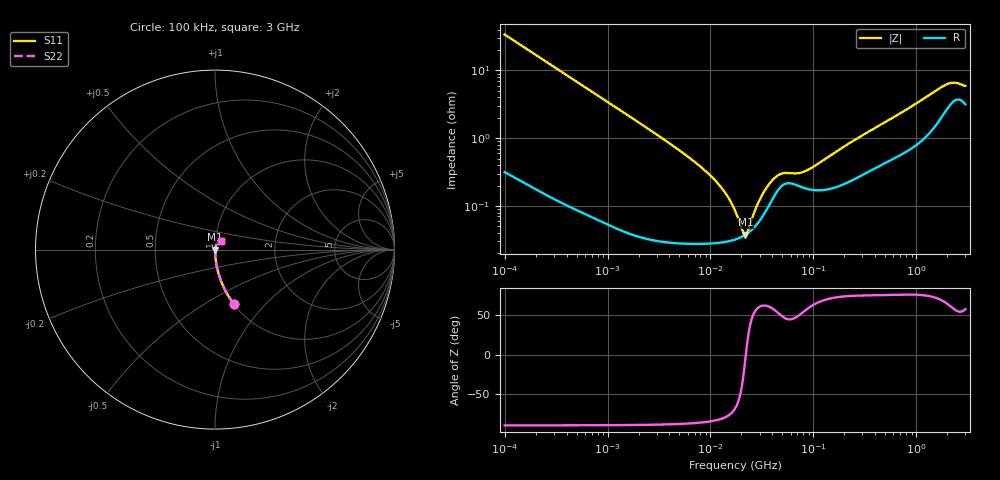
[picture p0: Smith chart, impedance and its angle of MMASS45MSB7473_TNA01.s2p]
! MMASS45MSB7473_TNA01  S-PARAMETER MODEL  ( Standard Model )
! Model Generated by TAIYO YUDEN Corporation (http://www.ty-top.com)
! Version 1.0
! TAIYO YUDEN Control No. 220601
! Copyright(c) 2013 TAIYO YUDEN CO.,LTD. All Rights Reserved.
! Product Description (link to TY-COMPAS)
! https://ds.yuden.co.jp/TYCOMPAS/or/detail?pn=MMASS45MSB7473KTNA01&u=M
! Products Name : Multilayer Ceramic Capacitors
! Characteristics :
!  Capacitance : 0.047 [uF] , Rated Voltage : 630 [V] , TCC : X7R
!  Case Size : 4.5 x 3.2 / 0.177 x 0.126 [mm/inch] , Thickness : 2.5 / 0.098 [mm/inch]
!  (Conditions: Temperature = 25 [degC] , DC Bias Voltage = 0 [V])
! External Node Assignments :
!  1  o---| |---o  2
! GND o---------o GND
! Frequency Range : 100kHz  -  3GHz  [ 401 STEP ]
# MHZ S RI R 50
! Freq[MHz].  S11 Real  S11 Imag  S21 Real  S21 Imag  S12 Real  S12 Imag  S22 Real  S22 Imag
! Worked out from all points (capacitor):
!   401 points, 100 kHz to 3 GHz, reference 50 ohm
!   read as one part in series: C = 46.7 nF near 105.3 kHz
!   lowest |Z| = 37.7 mohm at 21.84 MHz (marker M1)
!   series resonance near 22.07 MHz, so ESL is about 1.1 nH
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0.1  0.1059 -0.3031  0.8941 0.3031  0.8941 0.3031  0.1059 -0.3031
0.228123  0.0234 -0.1461  0.9766 0.1461  0.9766 0.1461  0.0234 -0.1461
0.562235  0.00451 -0.0608  0.9955 0.0608  0.9955 0.0608  0.00451 -0.0608
3.161081  0.000416 -0.0107  0.9996 0.0107  0.9996 0.0107  0.000416 -0.0107
6.504802  0.0003 -0.00489  0.9997 0.00489  0.9997 0.00489  0.0003 -0.00489
10.34438  0.000287 -0.00265  0.9997 0.00265  0.9997 0.00265  0.000287 -0.00265
14.09348  0.000298 -0.00149  0.9997 0.00149  0.9997 0.00149  0.000298 -0.00149
17.7727  0.000324 -0.000713  0.9997 0.000713  0.9997 0.000713  0.000324 -0.000713
20.21703  0.000351 -0.000289  0.9996 0.000289  0.9996 0.000289  0.000351 -0.000289
21.84217  0.000375 -3.36e-05  0.9996 3.36e-05  0.9996 3.36e-05  0.000375 -3.36e-05
22.99754  0.000395 0.000139  0.9996 -0.000139  0.9996 -0.000139  0.000395 0.000139
27.54426  0.00051 0.000762  0.9995 -0.000762  0.9995 -0.000762  0.00051 0.000762
31.3325  0.000662 0.00123  0.9993 -0.00123  0.9993 -0.00123  0.000662 0.00123
35.64176  0.000917 0.00169  0.9991 -0.00169  0.9991 -0.00169  0.000917 0.00169
41.60216  0.0014 0.00214  0.9986 -0.00214  0.9986 -0.00214  0.0014 0.00214
49.82709  0.002 0.00226  0.998 -0.00226  0.998 -0.00226  0.002 0.00226
73.34282  0.00196 0.00236  0.998 -0.00236  0.998 -0.00236  0.00196 0.00236
97.38194  0.00173 0.00326  0.9983 -0.00326  0.9983 -0.00326  0.00173 0.00326
547.5153  0.00493 0.018  0.9951 -0.018  0.9951 -0.018  0.00493 0.018
1935.725  0.0276 0.0532  0.9724 -0.0532  0.9724 -0.0532  0.0276 0.0532
2318.426  0.0369 0.0522  0.9631 -0.0522  0.9631 -0.0522  0.0369 0.0522
3000  0.0329 0.0469  0.9671 -0.0469  0.9671 -0.0469  0.0329 0.0469
